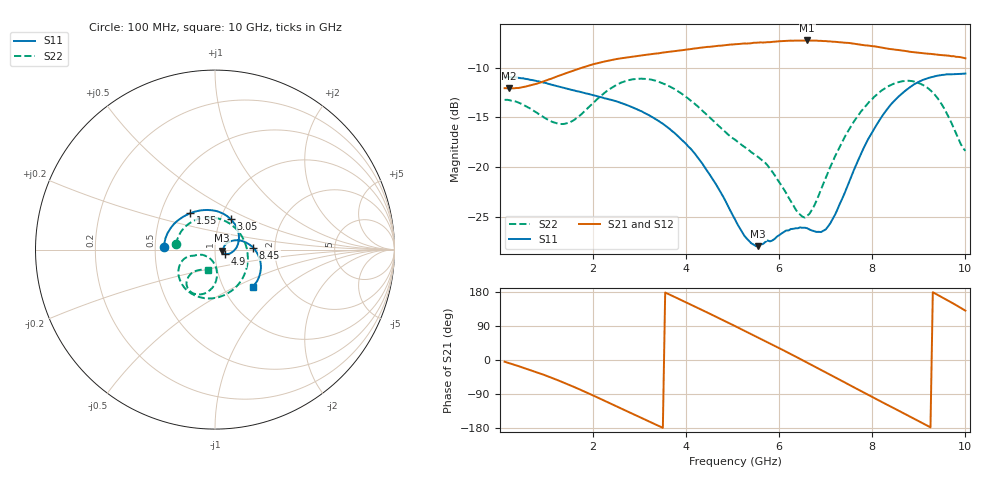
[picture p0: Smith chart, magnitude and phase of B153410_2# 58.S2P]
!  2-Port S-parameters saved by WinCal
! VAR MeasName=S-Parameters (CALIBRATED_DATA) read from VNA (N5245A)
! VAR MeasDate=2016-12-23 10:02:28
! VAR NAME=B153410_2# 58
! VAR FILENAME=B153410_2# 58.S2P
! VAR DATE=2016-12-23 10:02:28
! VAR PHYS_PORTS=1,2
# Hz S DB R 50
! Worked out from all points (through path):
!   199 points, 100 MHz to 10 GHz, reference 50 ohm
!   highest |S21| = -7.23 dB at 6.6 GHz (marker M1); lowest = -12.1 dB at 200 MHz (marker M2)
!   group delay of S21, straight-line fit = 167 ps
!   lowest |S11| = -28.0 dB at 5.55 GHz (marker M3), VSWR 1.08, Z = 54.1 - j0.669 ohm
!   |S11| at or under -10 dB: start of sweep to end of sweep
!   |S22| runs from -25.1 to -11.1 dB; largest |S21 - S12| = 0.004
!   S11 on the Smith chart (normalised r, x): 100 MHz: 0.56, +0.02; 1.55 GHz: 0.71, +0.30; 3.05 GHz: 1.12, +0.39; 4.9 GHz: 1.12, -0.06; 8.45 GHz: 1.54, +0.03; 10 GHz: 1.38, -0.62
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1e8  -10.95 176.7  -12.05 -4.5  -12.04 -4.6  -13.23 172.3
2e8  -10.93 172.8  -12.08 -8.5  -12.05 -8.5  -13.25 163.8
9e8  -11.45 146.5  -11.42 -37.2  -11.42 -37.3  -14.85 97.0
1.55e9  -12.23 123.9  -10.32 -69.0  -10.33 -69.1  -15.37 15.2
1.75e9  -12.45 116.9  -10.00 -79.7  -10.02 -79.8  -14.68 -9.4
2.45e9  -13.30 89.7  -9.15 -119.0  -9.18 -119.2  -11.87 -75.2
3.05e9  -14.39 62.0  -8.74 -153.4  -8.77 -153.4  -11.09 -113.7
3.4e9  -15.33 44.4  -8.54 -173.4  -8.55 -173.3  -11.38 -131.0
4.1e9  -18.16 7.6  -8.10 146.2  -8.10 146.4  -13.31 -156.0
4.9e9  -23.95 -23.1  -7.68 98.7  -7.68 98.7  -16.72 -165.5
5.05e9  -25.28 -24.2  -7.62 89.5  -7.63 89.7  -17.24 -165.3
5.55e9  -27.98 -8.9  -7.45 59.0  -7.44 59.2  -19.00 -163.8
6.1e9  -26.55 -1.1  -7.28 25.0  -7.29 25.1  -22.26 -158.2
6.6e9  -26.17 -2.4  -7.23 -6.8  -7.25 -6.8  -24.93 -118.7
6.7e9  -26.40 -0.4  -7.24 -13.3  -7.25 -13.3  -24.33 -108.3
7.05e9  -25.99 14.2  -7.33 -36.1  -7.34 -35.9  -20.55 -87.9
7.55e9  -20.95 28.8  -7.52 -68.5  -7.55 -68.4  -15.83 -86.9
7.95e9  -16.87 21.1  -7.78 -94.2  -7.80 -94.1  -13.34 -94.3
8.35e9  -13.99 6.7  -8.08 -120.0  -8.09 -119.7  -11.84 -104.9
8.45e9  -13.43 2.9  -8.13 -126.3  -8.15 -126.0  -11.62 -107.9
9.25e9  -10.96 -26.9  -8.59 -177.8  -8.61 -177.4  -12.27 -130.7
1e10  -10.57 -44.2  -9.03 130.3  -9.02 130.9  -18.36 -109.3
